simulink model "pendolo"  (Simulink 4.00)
settings: Solver=ode45  SolverMode=SingleTasking  StartTime=0.0  StopTime=Tf  FixedStep=Tc  MaxStep=Tc  RelTol=1e-3
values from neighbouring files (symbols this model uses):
  b = 10    [pendolo_control.m]
  g = 9.81    [pendolo_control.m]
  Kd = place(Ad,Bd,[p1 p2 p3 p4])    [pendolo_control.m]
  L = .5    (= 0.5)    [pendolo_control.m]
  m1 = .1    (= 0.1)    [pendolo_control.m]
  M2 = 2    [pendolo_control.m]
  Tc = .01    (= 0.01)    [pendolo_control.m]
  Var_v = [.0015 .005]'    [pendolo_control.m]
  Var_w = [.0001 .0001 .0001 .0001]    [pendolo_control.m]
  x0 = []    [pendan.m]    (also in pendolo_control.m = [.1 0 .1 0]')
undefined symbols (not defined in the file or in its folder): ekf
libraries: simulink3 x2

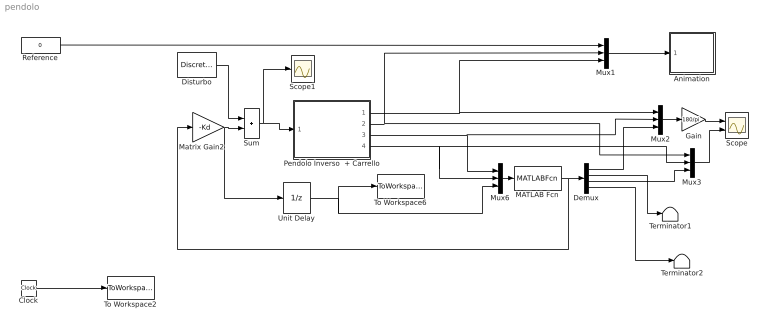
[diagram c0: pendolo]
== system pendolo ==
  Animation : Subsystem  mask(Pendulum plot){}
      mask help: Pendulum plot
      mask init:
      | RefBlock=&1;
  Clock : Clock
  Demux : Demux  Outputs=4  BusSelectionMode=off
  Disturbo : DiscretePulseGenerator  PulseType=Sample-based  Amplitude=80  Period=1500  PulseWidth=100  PhaseDelay=1000  SampleTime=Tc
  Gain : Gain  Gain=180/pi  Multiplication=Element-wise(K.*u)  SaturateOnIntegerOverflow=on
  MATLAB Fcn : MATLABFcn  MATLABFcn=ekf(u(1),u(2),u(3))  OutputDimensions=4  OutputSignalType=auto  Output1D=on
  Matrix Gain2 : Gain  Gain=-Kd  Multiplication=Matrix(K*u)  SaturateOnIntegerOverflow=on
  Mux{1..3,6} (4 alike) : Mux  Inputs=3
  Pendolo Inverso  + Carrello : Subsystem  mask{b=b, m1=m1, g=g, L=L, M2=M2}
      mask prompts: b "Coefficiente attrito (b)"; m1 "Massa del pendolo (m1)"; g "Accelerazione di gravita' (g)"; L "Lunghezza del pendolo (L)"; M2 "Massa del carrello (M2)"
  Reference : Constant  Value=0
  Scope : Scope  NumInputPorts=2
  Scope1 : Scope
  Sum : Sum  Inputs=|++  SaturateOnIntegerOverflow=on
  Terminator1 : Terminator
  Terminator2 : Terminator
  To Workspace2 : ToWorkspace  VariableName=T  SampleTime=Tc  SaveFormat=Array
  To Workspace6 : ToWorkspace  VariableName=u_d  SampleTime=Tc  SaveFormat=Array
  Unit Delay : UnitDelay  X0=0  SampleTime=Tc
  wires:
  Mux1/1 -> Animation/1(in_1)
  Reference/1 -> Mux1/1
  Mux2/1 -> Gain/1
  Clock/1 -> To Workspace2/1
  Mux3/1 -> Scope/2
  Matrix Gain2/1 -> Unit Delay/1, Sum/2
  Mux6/1 -> MATLAB Fcn/1
  Pendolo Inverso  + Carrello/4(z) -> Mux6/2, Mux3/2
  Pendolo Inverso  + Carrello/3(Theta) -> Mux6/1, Mux2/2
  Unit Delay/1 -> To Workspace6/1, Mux6/3
  Pendolo Inverso  + Carrello/2(z_nf) -> Mux1/2, Mux3/1
  Pendolo Inverso  + Carrello/1(Theta_nf) -> Mux1/3, Mux2/1
  Demux/3 -> Mux3/3
  Demux/1 -> Mux2/3
  Sum/1 -> Scope1/1, Pendolo Inverso  + Carrello/1(Forza)
  Disturbo/1 -> Sum/1
  Gain/1 -> Scope/1
  MATLAB Fcn/1 -> Demux/1, Matrix Gain2/1
  Demux/2 -> Terminator1/1
  Demux/4 -> Terminator2/1

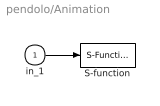
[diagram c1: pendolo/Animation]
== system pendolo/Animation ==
  in_1 : Inport  Port=1  LatchInput=off
  S-function : S-Function  FunctionName=pendan  Parameters=RefBlock  PortCounts=[]  SFunctionModules=''
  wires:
  in_1/1 -> S-function/1

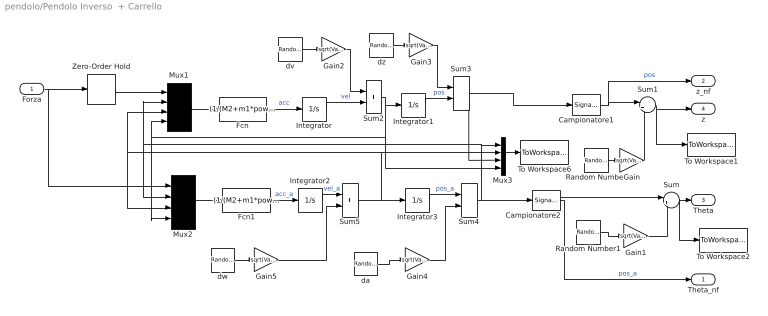
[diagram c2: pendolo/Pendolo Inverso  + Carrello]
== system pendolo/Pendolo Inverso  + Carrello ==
  Forza : Inport  Port=1  LatchInput=off
  Campionatore1 : simulink3/Signals & Systems/Signal Specification  D=-1  Ts=Tc  DataType=auto
  Campionatore2 : simulink3/Signals & Systems/Signal Specification  D=-1  Ts=Tc  DataType=auto
  Fcn : Fcn  Expr=(1/(M2+m1*power(sin(u(2)),2)))*(m1*L*sin(u(2))*power(u(3),2)-m1*g*sin(u(2))*cos(u(2))+u(1)-b*u(4))
  Fcn1 : Fcn  Expr=(1/(M2+m1*power(sin(u(2)),2)))*((M2+m1)/L*g*sin(u(2))-m1*sin(u(2))*cos(u(2))*power(u(3),2)-(u(1)-b*u(4))/L*cos(u(2)))
  Gain : Gain  Gain=sqrt(Var_v(2))  Multiplication=Element-wise(K.*u)  SaturateOnIntegerOverflow=on
  Gain1 : Gain  Gain=sqrt(Var_v(1))  Multiplication=Element-wise(K.*u)  SaturateOnIntegerOverflow=on
  Gain2 : Gain  Gain=sqrt(Var_w(4))  Multiplication=Element-wise(K.*u)  SaturateOnIntegerOverflow=on
  Gain3 : Gain  Gain=sqrt(Var_w(3))  Multiplication=Element-wise(K.*u)  SaturateOnIntegerOverflow=on
  Gain4 : Gain  Gain=sqrt(Var_w(1))  Multiplication=Element-wise(K.*u)  SaturateOnIntegerOverflow=on
  Gain5 : Gain  Gain=sqrt(Var_w(2))  Multiplication=Element-wise(K.*u)  SaturateOnIntegerOverflow=on
  Integrator : Integrator  ExternalReset=none  InitialConditionSource=internal  InitialCondition=x0(4)  LimitOutput=off  UpperSaturationLimit=inf  LowerSaturationLimit=-inf  ShowSaturationPort=off  ShowStatePort=off  AbsoluteTolerance=auto
  Integrator1 : Integrator  ExternalReset=none  InitialConditionSource=internal  InitialCondition=x0(3)  LimitOutput=off  UpperSaturationLimit=inf  LowerSaturationLimit=-inf  ShowSaturationPort=off  ShowStatePort=off  AbsoluteTolerance=auto
  Integrator2 : Integrator  ExternalReset=none  InitialConditionSource=internal  InitialCondition=x0(2)  LimitOutput=off  UpperSaturationLimit=inf  LowerSaturationLimit=-inf  ShowSaturationPort=off  ShowStatePort=off  AbsoluteTolerance=auto
  Integrator3 : Integrator  ExternalReset=none  InitialConditionSource=internal  InitialCondition=x0(1)  LimitOutput=off  UpperSaturationLimit=inf  LowerSaturationLimit=-inf  ShowSaturationPort=off  ShowStatePort=off  AbsoluteTolerance=auto
  Mux1 : Mux  Inputs=4
  Mux2 : Mux  Inputs=4
  Mux3 : Mux  Inputs=4
  Random Number : RandomNumber  Mean=0  Variance=1  Seed=ceil(3522*rand)  SampleTime=Tc
  Random Number1 : RandomNumber  Mean=0  Variance=1  Seed=ceil(4234*rand)  SampleTime=Tc
  Sum{,1..5} (6 alike) : Sum  Inputs=|++  SaturateOnIntegerOverflow=on
  To Workspace1 : ToWorkspace  VariableName=z_m  SampleTime=Tc  SaveFormat=Array
  To Workspace2 : ToWorkspace  VariableName=theta_m  SampleTime=Tc  SaveFormat=Array
  To Workspace6 : ToWorkspace  VariableName=x_real  SampleTime=Tc  SaveFormat=Array
  Zero-Order Hold : ZeroOrderHold  SampleTime=Tc
  da : RandomNumber  Mean=0  Variance=1  Seed=ceil(2341*rand)  SampleTime=Tc
  dv : RandomNumber  Mean=0  Variance=1  Seed=ceil(1000*rand)  SampleTime=Tc
  dw : RandomNumber  Mean=0  Variance=1  Seed=ceil(4322*rand)  SampleTime=Tc
  dz : RandomNumber  Mean=0  Variance=1  Seed=ceil(8961*rand)  SampleTime=Tc
  Theta_nf : Outport  Port=1
  z_nf : Outport  Port=2
  Theta : Outport  Port=3
  z : Outport  Port=4
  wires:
  Fcn/1 -> Integrator/1  "acc"
  Forza/1 -> Mux2/1, Zero-Order Hold/1
  Mux1/1 -> Fcn/1
  Fcn1/1 -> Integrator2/1  "acc_a"
  Mux2/1 -> Fcn1/1
  Random Number/1 -> Gain/1
  Sum1/1 -> z/1, To Workspace1/1
  Sum/1 -> Theta/1, To Workspace2/1
  Random Number1/1 -> Gain1/1
  Gain/1 -> Sum1/2
  Gain1/1 -> Sum/2
  Campionatore2/1 -> Sum/1, Theta_nf/1  "pos_a"
  Zero-Order Hold/1 -> Mux1/1
  Mux3/1 -> To Workspace6/1
  Integrator/1 -> Sum2/2  "vel"
  dv/1 -> Gain2/1
  Gain2/1 -> Sum2/1
  Sum2/1 -> Integrator1/1, Mux1/4, Mux2/4, Mux3/4
  Campionatore1/1 -> Sum1/1, z_nf/1  "pos"
  Integrator1/1 -> Sum3/2  "pos"
  dz/1 -> Gain3/1
  Gain3/1 -> Sum3/1
  Sum3/1 -> Campionatore1/1, Mux3/3
  da/1 -> Gain4/1
  Gain4/1 -> Sum4/2
  Integrator3/1 -> Sum4/1  "pos_a"
  Sum4/1 -> Campionatore2/1, Mux3/1, Mux1/2, Mux2/2
  dw/1 -> Gain5/1
  Gain5/1 -> Sum5/2
  Integrator2/1 -> Sum5/1  "vel_a"
  Sum5/1 -> Integrator3/1, Mux2/3, Mux1/3, Mux3/2
